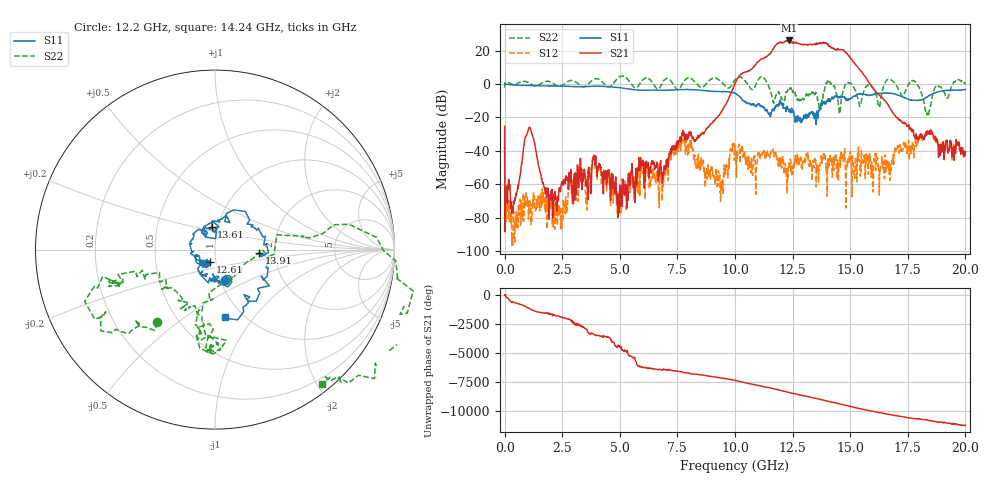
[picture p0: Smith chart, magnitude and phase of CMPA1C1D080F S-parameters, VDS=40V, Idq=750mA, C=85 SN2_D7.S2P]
!Keysight Technologies,E5071C,MY46632380,B.14.03
!Date: Tue Nov 10 05:42:26 2020
!Data & Calibration Information:
!Freq	S11:SOLT2(ON)	S21:SOLT2(ON)	S12:SOLT2(ON)	S22:SOLT2(ON)
!PortZ  Port1:50+j0  Port2:50+j0
!Above PortZ is port z conversion or system Z0 setting when saving the data.
!When reading, reference impedance value at option line is always used.
# Hz S dB R 50
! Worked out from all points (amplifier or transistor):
!   1601 points, 300 kHz to 20 GHz, reference 50 ohm
!   highest |S21| = 26.1 dB at 12.35 GHz (marker M1)
!   |S21| within 3 dB of that: 11.76 GHz to 14.05 GHz (2.292 GHz wide, 17.8 % of centre)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
!   unconditionally stable (mu >= 1): 11.44 GHz to 13.91 GHz; 15.06 GHz to 16.49 GHz; 17.89 GHz to 19.46 GHz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
!   at 3.325 GHz: K = 5886.04, MAG = -40.9 dB, |S12| = -51.4 dB
!   at 10 GHz: K = -25.67, MSG = 19.8 dB, |S12| = -39.3 dB
!   at 20 GHz: K = 66.22, MAG = -21.7 dB, |S12| = -39.6 dB
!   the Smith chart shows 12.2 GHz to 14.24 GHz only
!   S11 on the Smith chart (normalised r, x): 12.2 GHz: 1.05, -0.37; 12.61 GHz: 0.94, -0.13; 13.61 GHz: 0.93, +0.24; 13.91 GHz: 1.65, -0.06; 14.24 GHz: 0.83, -0.73
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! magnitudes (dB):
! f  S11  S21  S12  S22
! 300 kHz  0.1  -25.3  -35.5  -2.1
! 387.8 MHz  -0.6  -70.0  -76.3  -0.3
! 1.063 GHz  -0.9  -26.1  -69.9  0.7
! 2.013 GHz  -1.2  -67.2  -65.2  1.1
! 3.338 GHz  -1.6  -51.2  -50.3  -1.4
! 3.9 GHz  -1.4  -45.2  -46.3  3.1
! 5 GHz  -2.2  -60.5  -66.3  4.4
! 6.675 GHz  -3.7  -58.0  -60.2  -3.0
! 7.7 GHz  -3.3  -30.0  -33.4  -0.3
! 9.4 GHz  -4.5  -16.6  -58.1  1.5
! 10 GHz  -5.5  0.3  -39.3  2.5
! 12.2 GHz  -15.0  25.5  -52.2  -5.7
! 12.35 GHz  -16.4  26.1  -47.1  -2.1
! 12.61 GHz  -22.9  25.2  -42.9  -5.1
! 13.34 GHz  -17.2  23.5  -48.2  -5.5
! 13.61 GHz  -17.9  24.1  -48.3  -11.2
! 13.91 GHz  -12.2  24.6  -42.5  -0.9
! 14.24 GHz  -8.4  21.4  -51.2  -0.4
! 16.25 GHz  -5.6  -6.6  -55.1  -14.0
! 16.68 GHz  -5.4  -13.1  -46.8  2.9
! 18.35 GHz  -7.6  -28.3  -28.5  -17.4
! 20 GHz  -3.3  -40.6  -39.6  -0.1
